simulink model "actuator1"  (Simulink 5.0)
settings: Solver=ode45  StartTime=0.0  StopTime=.35  MaxStep=1e-4  RelTol=1e-3

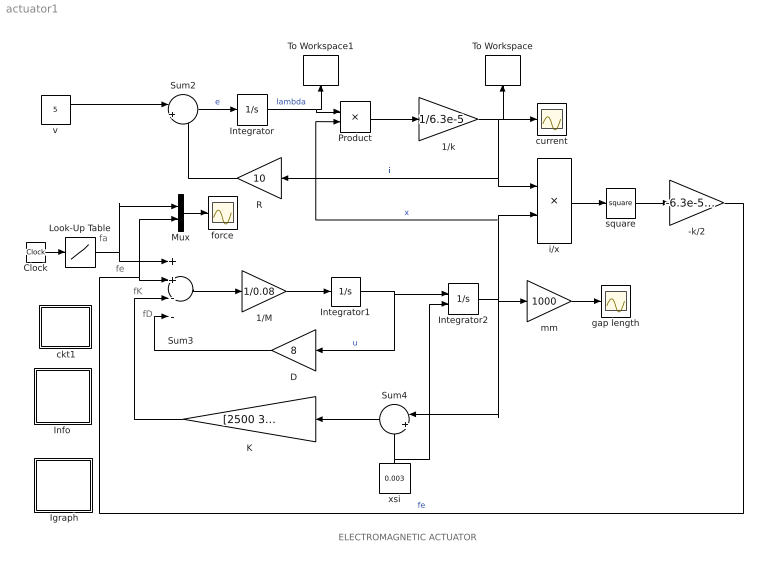
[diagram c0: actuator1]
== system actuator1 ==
  note: ELECTROMAGNETIC ACTUATOR
  note: fe
  note: fa
  note: fK
  note: fD
  " Igraph" : Subsystem
  " ckt1" : Subsystem
  -k/2 : Gain  Gain=-6.3e-5/2
  1/M : Gain  Gain=1/0.08
  1/k : Gain  Gain=1/6.3e-5
  Clock : Clock
  D : Gain  Orientation=left  Gain=8
  Info : Subsystem
  Integrator : Integrator
  Integrator1 : Integrator
  Integrator2 : Integrator  InitialConditionSource=external  InitialCondition=0.003
  K : Gain  Orientation=left  Gain=[2500 3000 3500]
  Look-Up Table : Lookup  InputValues=[0 0.1 0.1 0.25 0.25 1]  OutputValues=[0 0 4 4 0 0]
  Mux : Mux  Inputs=2
  Product : Product
  R : Gain  Orientation=left  Gain=10
  Sum2 : Sum  Inputs=|+-
  Sum3 : Sum  Inputs=++--
  Sum4 : Sum  Orientation=left  Inputs=|+-
  To Workspace : ToWorkspace  VariableName=i  SampleTime=-1  SaveFormat=Array
  To Workspace1 : ToWorkspace  VariableName=lambda  SampleTime=-1  SaveFormat=Array
  current : Scope
  force : Scope
  gap length : Scope
  i/x : Product  Inputs=*/
  mm : Gain  Gain=1000
  square : Math  Operator=square
  v : Constant  Value=5
  xsi : Constant  Orientation=up  Value=0.003
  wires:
  R/1 -> Sum2/2
  v/1 -> Sum2/1
  Sum2/1 -> Integrator/1  "e"
  Product/1 -> 1/k/1
  Sum3/1 -> 1/M/1
  D/1 -> Sum3/4
  K/1 -> Sum3/3
  square/1 -> -k/2/1
  1/k/1 -> i/x/1, R/1, current/1, To Workspace/1  "i"
  1/M/1 -> Integrator1/1
  i/x/1 -> square/1
  xsi/1 -> Sum4/2, Integrator2/2
  Sum4/1 -> K/1
  Mux/1 -> force/1
  -k/2/1 -> Sum3/2, Mux/2  "fe"
  Integrator/1 -> Product/1, To Workspace1/1  "lambda"
  Integrator1/1 -> D/1, Integrator2/1  "u"
  Look-Up Table/1 -> Sum3/1, Mux/1
  Clock/1 -> Look-Up Table/1
  Integrator2/1 -> Sum4/1, Product/2, i/x/2, mm/1  "x"
  mm/1 -> gap length/1

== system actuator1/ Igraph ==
  note: This demo simulates the running of an induction motor
  note: Double click the block to enter the machine parameters and initial conditions and start the simulation

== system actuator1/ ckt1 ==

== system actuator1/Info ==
  note: This demonstration illustrates the dynamic performance of an electromagnetic actuator modeled by a position-dependent inductance expressed by L(x) = k/x. Electrical system: v = Ri + d(lambda)/dt ; lambda = L(x) i or i = lambda* x / k Mechanical system: fa = Mdu/dt + Du + K(x-xsi) - fe ; fe = 0.5 i^2 dL/dx = -0.5*k*(i / x)^2 xsi = equilibrium position when i = 0 and fa = 0
  note: Electromagnetic actuator
  note: Double click following the simulation
